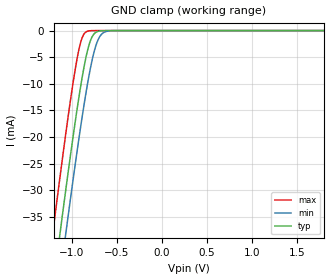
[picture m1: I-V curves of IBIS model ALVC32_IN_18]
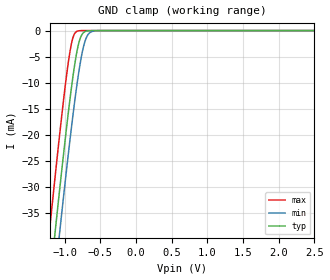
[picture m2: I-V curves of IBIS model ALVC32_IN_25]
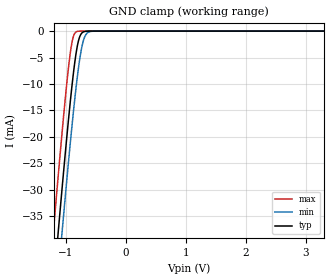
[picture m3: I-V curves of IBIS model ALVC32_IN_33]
| TEXAS INSTRUMENTS INCORPORATED
| Standard Linear and Logic Group
| IBIS Model of SN74ALVC32
| QUADRUPLE 2-INPUT POSITIVE-OR GATE
| This file contains package information for the following:
|  SOIC 14-pin (D) package as [Component] ALVC32_D
|  TVSOP 14-pin (DGV) package as [Component] ALVC32_DGV
|  TSSOP 14-pin (PW) package as [Component] ALVC32_PW
| This device can be powered at the following Vccs:
|  1.8 volt Vcc
|  2.5 volt Vcc
|  3.3 volt Vcc
| This file provides unique models under the [Model Selector] for each Vcc.
| For operation at a specific Vcc, select the appropriate model after each
| [Model Selector] keyword.
[IBIS Ver]   3.2
[Comment char]  |_char
[File Name]   sn74alvc32.ibs
[File Rev]   1.1 | a_die
[Date]   May 6, 2002
[Source]   Data created from TI-SPICE simulations at TI-SLL.
[Notes]   The following is an IBIS list for the ALVC32.
   Please contact sllibis@ti.com with questions and
   comments concerning SLL IBIS models.
   - We removed Power_Clamp curve from the input models
   since there is no power clamp diode there.
[Disclaimer] Property of Texas Instruments Incorporated.  Unauthorized
   reproduction and/or distribution is strictly prohibited.
   This product is protected under copyright law.
   Created  2002, (C) Copyright  2002, Texas Instruments
   Incorporated, All Rights Reserved
   UNLESS THERE IS A SIGNED, WRITTEN AGREEMENT TO THE
   CONTRARY, TEXAS INSTRUMENTS (TI) IS PROVIDING THE IBIS
   MODELS  AND WITHOUT ANY WARRANTY, EXPRESSED OR
   IMPLIED.  TI assumes no liability for:
   1) the accuracy of the IBIS models provided to your
   company;
   2) the proper functioning of these IBIS Models in your
   design or for any resulting applications; or
   3) infringement of patents, copyrights or intellectual
   property rights resulting from your use of these IBIS
   models.
   TI provides IBIS Models as a service to our customers.
   You and your company shall not distribute, sell or give
   these models to anyone else without prior written
   permission from TI.
   TI reserves the right to make changes to our products or
   to discontinue any semiconductor product or service
   without notice, and advises our customers to obtain the
   latest version of relevant information to verify, before
   placing orders, that the information being relied on is
   current.
   Please be aware that your receipt and use of the IBIS
   information provided shall serve as acceptance of these
   terms and conditions.  If you do not accept these terms,
   you should return or destroy the IBIS models and any
   other accompanying information immediately.
| Component ALVC32_D 14-pin SOIC
[Component]   ALVC32_D
[Manufacturer]   Texas Instruments, Inc.
[Package]
|   typ   min   max
R_pkg   3.100e-02   2.800e-02   3.400e-02
L_pkg   3.109e-09   2.462e-09   3.889e-09
C_pkg   4.730e-13   3.630e-13   6.280e-13
[Pin]   signal_name   model_name   R_pin   L_pin   C_pin
1   1A   ALVC32_IN   3.300e-02   3.854e-09   6.220e-13
2   1B   ALVC32_IN   3.200e-02   3.188e-09   4.730e-13
3   1Y   ALVC32_OUT   2.800e-02   2.462e-09   3.770e-13
4   2A   ALVC32_IN   3.100e-02   2.596e-09   3.630e-13
5   2B   ALVC32_IN   2.800e-02   2.521e-09   3.720e-13
6   2Y   ALVC32_OUT   3.400e-02   3.250e-09   4.760e-13
7   GND   GND   3.400e-02   3.889e-09   6.280e-13
8   3Y   ALVC32_OUT   3.400e-02   3.889e-09   6.280e-13
9   3A   ALVC32_IN   3.400e-02   3.250e-09   4.760e-13
10   3B   ALVC32_IN   2.800e-02   2.521e-09   3.720e-13
11   4Y   ALVC32_OUT   3.100e-02   2.596e-09   3.640e-13
12   4A   ALVC32_IN   2.800e-02   2.462e-09   3.770e-13
13   4B   ALVC32_IN   3.200e-02   3.188e-09   4.730e-13
14   VCC   POWER   3.300e-02   3.854e-09   6.220e-13
| Component ALVC32_DGV 14-pin TVSOP
[Component]   ALVC32_DGV
[Manufacturer]   Texas Instruments, Inc.
[Package]
|   typ   min   max
R_pkg   3.500e-02   2.000e-02   4.500e-02
L_pkg   2.499e-09   2.077e-09   2.966e-09
C_pkg   3.610e-13   3.050e-13   4.160e-13
[Pin]   signal_name   model_name   R_pin   L_pin   C_pin
1   1A   ALVC32_IN   2.700e-02   2.717e-09   3.730e-13
2   1B   ALVC32_IN   3.700e-02   2.434e-09   3.980e-13
3   1Y   ALVC32_OUT   3.400e-02   2.200e-09   3.160e-13
4   2A   ALVC32_IN   2.000e-02   2.077e-09   3.090e-13
5   2B   ALVC32_IN   3.000e-02   2.147e-09   3.050e-13
6   2Y   ALVC32_OUT   4.200e-02   2.580e-09   4.080e-13
7   GND   GND   3.900e-02   2.921e-09   3.850e-13
8   3Y   ALVC32_OUT   3.300e-02   2.841e-09   3.800e-13
9   3A   ALVC32_IN   4.200e-02   2.611e-09   4.100e-13
10   3B   ALVC32_IN   3.800e-02   2.331e-09   3.290e-13
11   4Y   ALVC32_OUT   2.600e-02   2.223e-09   3.190e-13
12   4A   ALVC32_IN   3.400e-02   2.259e-09   3.130e-13
13   4B   ALVC32_IN   4.500e-02   2.681e-09   4.160e-13
14   VCC   POWER   4.200e-02   2.966e-09   3.860e-13
| Component ALVC32_PW 14-pin TSSOP
[Component]   ALVC32_PW
[Manufacturer]   Texas Instruments, Inc.
[Package]
|   typ   min   max
R_pkg   3.200e-02   2.900e-02   3.500e-02
L_pkg   2.378e-09   2.170e-09   2.680e-09
C_pkg   3.140e-13   2.700e-13   3.350e-13
[Pin]   signal_name   model_name   R_pin   L_pin   C_pin
1   1A   ALVC32_IN   3.300e-02   2.618e-09   3.300e-13
2   1B   ALVC32_IN   3.100e-02   2.313e-09   3.170e-13
3   1Y   ALVC32_OUT   3.000e-02   2.310e-09   3.140e-13
4   2A   ALVC32_IN   3.100e-02   2.173e-09   2.720e-13
5   2B   ALVC32_IN   3.000e-02   2.204e-09   3.090e-13
6   2Y   ALVC32_OUT   3.200e-02   2.315e-09   3.170e-13
7   GND   GND   3.500e-02   2.680e-09   3.350e-13
8   3Y   ALVC32_OUT   3.300e-02   2.640e-09   3.330e-13
9   3A   ALVC32_IN   3.400e-02   2.347e-09   3.190e-13
10   3B   ALVC32_IN   2.900e-02   2.277e-09   3.130e-13
11   4Y   ALVC32_OUT   3.100e-02   2.170e-09   2.700e-13
12   4A   ALVC32_IN   3.100e-02   2.244e-09   3.110e-13
13   4B   ALVC32_IN   3.300e-02   2.343e-09   3.210e-13
14   VCC   POWER   3.500e-02   2.657e-09   3.320e-13
| Model ALVC32_IN
[Model Selector]   ALVC32_IN
ALVC32_IN_18   1.8 volt Vcc
ALVC32_IN_25   2.5 volt Vcc
ALVC32_IN_33   3.3 volt Vcc
| Model ALVC32_OUT
[Model Selector]   ALVC32_OUT
ALVC32_OUT_18   1.8 volt Vcc
ALVC32_OUT_25   2.5 volt Vcc
ALVC32_OUT_33   3.3 volt Vcc
| Models and submodels in the file (6): ALVC32_IN_18 (Input), ALVC32_IN_25 (Input), ALVC32_IN_33 (Input), ALVC32_OUT_18 (Output), ALVC32_OUT_25 (Output), ALVC32_OUT_33 (Output)
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[Model]   ALVC32_IN_18
Model_type  Input
Vinl=0.5775
Vinh=1.2675
| variable   typ   min   max
C_comp   3.95pF   3.41pF   4.64pF
[Temperature Range]   40   100   -40
| Ambient temperature   25   85   -40
[Voltage range]   1.8   1.65   1.95
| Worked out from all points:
|   GND clamp passes 1 mA (typ) near -0.77 V on its own axis
[GND Clamp]
| ALVC32_IN_18
|   Voltage   I(typ)   I(min)   I(max)
-1.8V     -129.8mA   -137.8mA   -119.7mA
-1.205V   -48.27mA   -56.56mA   -37.63mA
-1.125V   -37.77mA   -46.06mA   -27.13mA
-1.06V    -29.44mA   -37.69mA   -18.89mA
-980mV    -19.61mA   -27.69mA   -9.485mA
-925mV    -13.29mA   -21.11mA   -4.122mA
-880mV    -8.606mA   -15.99mA   -1.263mA
-835mV    -4.656mA   -11.25mA   -214.1uA
-780mV    -1.472mA   -6.227mA   -17.15uA
-725mV    -285.9uA   -2.596mA   -1.294uA
-615mV    -6.479uA   -167.8uA   -7.305nA
1.8V      3.326pA    6.142pA    3.026pA
[Model]   ALVC32_IN_25
Model_type  Input
Vinl=0.7
Vinh=1.7
| variable   typ   min   max
C_comp   3.90pF   3.10pF   4.62pF
[Temperature Range]   40   100   -40
| Ambient temperature   25   85   -40
[Voltage range]   2.5   2.3   2.7
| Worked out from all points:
|   GND clamp passes 1 mA (typ) near -0.77 V on its own axis
[GND Clamp]
| ALVC32_IN_25
|   Voltage   I(typ)   I(min)   I(max)
-2.5V     -228.1mA   -235.8mA   -218.5mA
-1.23V    -51.59mA   -59.87mA   -40.97mA
-1.2V     -47.61mA   -55.9mA    -36.97mA
-1.13V    -38.42mA   -46.71mA   -27.77mA
-1.07V    -30.71mA   -38.96mA   -20.13mA
-925mV    -13.29mA   -21.11mA   -4.122mA
-880mV    -8.606mA   -15.99mA   -1.263mA
-830mV    -4.281mA   -10.75mA   -171.6uA
-780mV    -1.472mA   -6.227mA   -17.15uA
-720mV    -242.5uA   -2.354mA   -1.023uA
-600mV    -3.832uA   -109.2uA   -3.608nA
2.5V      4.713pA    7.577pA    4.389pA
[Model]   ALVC32_IN_33
Model_type  Input
Vinl=0.8
Vinh=2.0
| variable   typ   min   max
C_comp   3.87pF   2.95pF   5.06pF
[Temperature Range]   40   100   -40
| Ambient temperature   25   85   -40
[Voltage range]   3.3   3   3.6
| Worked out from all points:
|   GND clamp passes 1 mA (typ) near -0.77 V on its own axis
[GND Clamp]
| ALVC32_IN_33
|   Voltage   I(typ)   I(min)   I(max)
-3.3V     -341.5mA   -348.9mA   -332.3mA
-1.215V   -49.6mA    -57.88mA   -38.96mA
-1.185V   -45.62mA   -53.91mA   -34.98mA
-1.125V   -37.77mA   -46.06mA   -27.13mA
-1.065V   -30.08mA   -38.33mA   -19.51mA
-920mV    -12.75mA   -20.53mA   -3.718mA
-875mV    -8.124mA   -15.45mA   -1.065mA
-825mV    -3.922mA   -10.26mA   -137.1uA
-775mV    -1.291mA   -5.83mA    -13.57uA
-715mV    -205.4uA   -2.128mA   -808.5nA
-585mV    -2.266uA   -70.82uA   -1.783nA
3.3V      6.304pA    9.258pA    5.93pA
